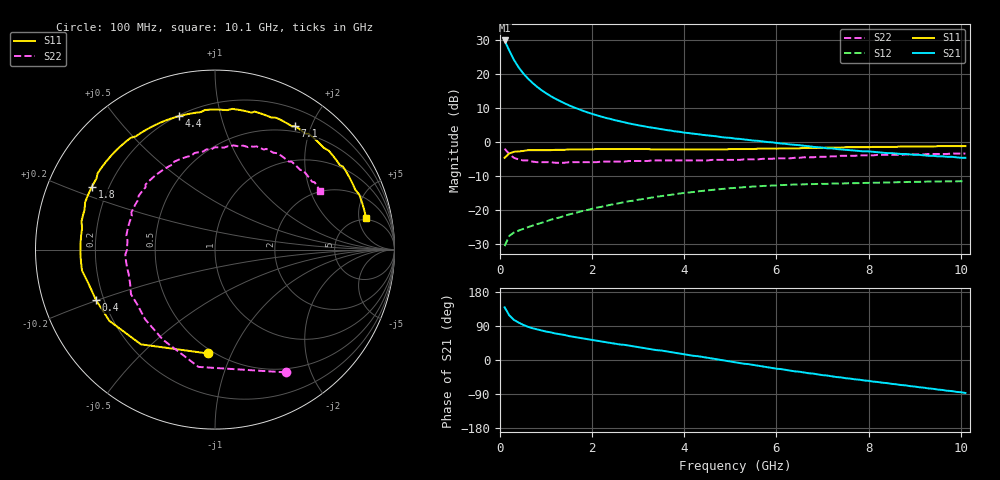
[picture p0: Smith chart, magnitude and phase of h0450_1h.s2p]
!HBFP-0450
!S and NOISE PARAMETERS at Vce=1V  Ic=50mA.  LAST UPDATED  09-04-98
# GHZ S MA R  50
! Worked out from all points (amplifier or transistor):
!   101 points, 100 MHz to 10.1 GHz, reference 50 ohm
!   highest |S21| = 29.8 dB at 100 MHz (marker M1)
!   |S21| within 3 dB of that: start of sweep to 202.3 MHz
!   unconditionally stable (mu >= 1): 2.194 GHz to end of sweep
!   at 1.7 GHz: K = 0.95, MSG = 15.2 dB, |S12| = -20.7 dB
!   at 5.1 GHz: K = 1.09, MAG = 5.4 dB, |S12| = -13.6 dB
!   at 10.1 GHz: K = 1.09, MAG = 1.6 dB, |S12| = -11.7 dB
!   lowest NFmin = 1.74 dB at 1.8 GHz
!   S11 on the Smith chart (normalised r, x): 100 MHz: 0.47, -0.82; 400 MHz: 0.17, -0.20; 1.8 GHz: 0.14, +0.24; 4.4 GHz: 0.20, +0.75; 7.1 GHz: 0.42, +1.77; 10.1 GHz: 4.55, +6.25
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0.1  0.58 -94.0  30.94 139.0  0.029 56.0  0.79 -60.0
0.2  0.67 -128.0  22.06 118.0  0.041 42.0  0.66 -98.0
0.3  0.71 -146.0  16.15 106.0  0.046 35.0  0.58 -120.0
0.4  0.72 -157.0  12.56 99.0  0.049 33.0  0.55 -135.0
0.5  0.73 -165.0  10.22 93.0  0.052 33.0  0.53 -145.0
0.6  0.75 -171.0  8.61 88.0  0.055 32.0  0.53 -152.0
0.7  0.75 -175.0  7.39 84.0  0.058 33.0  0.51 -158.0
0.8  0.75 -179.0  6.47 81.0  0.061 34.0  0.5 -164.0
0.9  0.75 177.0  5.74 78.0  0.064 35.0  0.5 -169.0
1.1  0.75 171.0  4.69 73.0  0.071 36.0  0.5 -177.0
1.3  0.76 165.0  3.97 68.0  0.077 36.0  0.49 177.0
1.5  0.77 160.0  3.43 63.0  0.085 36.0  0.5 171.0
1.8  0.77 153.0  2.85 57.0  0.096 35.0  0.5 164.0
2.1  0.78 147.0  2.45 51.0  0.107 34.0  0.5 158.0
2.5  0.78 139.0  2.07 43.0  0.121 31.0  0.51 150.0
3.5  0.77 121.0  1.53 25.0  0.158 21.0  0.53 134.0
4.4  0.77 105.0  1.26 8.0  0.189 9.0  0.53 118.0
5.1  0.78 92.0  1.11 -6.0  0.209 -2.0  0.54 106.0
6.8  0.81 62.0  0.84 -36.0  0.238 -27.0  0.59 77.0
7.1  0.82 57.0  0.8 -41.0  0.24 -31.0  0.6 72.0
8.5  0.84 36.0  0.68 -63.0  0.252 -50.0  0.64 53.0
10.1  0.86 12.0  0.58 -87.0  0.261 -72.0  0.67 29.0
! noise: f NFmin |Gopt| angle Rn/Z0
1.8  1.74  0.627  -152  0.09
2  1.77  0.628  -149  0.11
2.5  1.87  0.641  -139  0.17
3.5  2.15  0.669  -122  0.35
4  2.31  0.685  -112  0.52
5  2.53  0.712  -93  0.91
5.5  2.66  0.731  -83  1.26
7  3.04  0.77  -56  2.39
8  3.35  0.788  -40  3.31
10  3.8  0.809  -12  4.9
